| IBIS file stm32u595_599_5a5_5a9_wlcsp208_dsi_smps.ibs
[IBIS ver] 4.2
[File name] stm32u595_599_5a5_5a9_wlcsp208_dsi_smps.ibs
[File Rev] rev2.0
[Date]  11-09-2023
[Source] Data Created at STMicroelectronics
[Notes]  File originated from ELDO simulations.
[Disclaimer]  This information is for modeling purpose only and is
   not guaranteed. The information is subject to change without
   notice.
[Copyright] Copyright 2023 STMicroelectronics Inc.
|   Component stm32u595_599_5a5_5a9_wlcsp208_dsi_smps
[Component] stm32u595_599_5a5_5a9_wlcsp208_dsi_smps
[Manufacturer] STMicroelectronics
[Package]
| variable   typ   min   max
R_pkg  0  NA  NA
L_pkg  0  NA  NA
C_pkg  0  NA  NA
[Pin]   signal_name   model_name
A2  VDDUSB  power
A4  VDD11  nc
A6  VDD  power
A8  PA15  nc
A10  PD1  io8_100m_hslv_ft
A12  VDD  power
A14  PG13  io8_100m_hslv_ft
A16  VDDIO2  power
A18  PB6  io8_100m_i2c_ft
A20  PE0  io8_100m_hslv_ft
A22  VD11  nc
A24  VDD  power
A26  VDD  power
B1  PA12  io8_100m_ft
B3  PA13  io8_100m_ft
B5  VSS  gnd
B7  PH2  io8_100m_hslv_ft
B9  PC10  io8_100m_ft
B11  VSS  gnd
B13  PG9  io8_100m_hslv_ft
B15  VSS  gnd
B17  PB3  io8_100m_i2c_ft
B19  PB8  io8_100m_i2c_ft
B21  PE1  io8_100m_hslv_ft
B23  VSS  gnd
B25  VBAT  power
C2  PA11  io8_100m_ft
C4  PA10  io8_100m_usb_id
C6  PA9  io8_100m_usb_vbus_ft
C8  PA8  io8_166m_hslv_ft
C10  PC11  io8_100m_hslv_ft
C12  PD3  io8_166m_hslv_ft
C14  PD7  io8_100m_hslv_ft
C16  PG14  io8_100m_hslv_ft
C18  PB5  io8_166m_hslv_ft
C20  PB9  io8_100m_i2c_ft
C22  PI5  io8_100m_hslv_ft
C24  PE6  io8_100m_hslv_tamp_ft
C26  PC14-OSC32_IN  nc
D1  VDD11USB  nc
D3  PC7  io8_100m_ft
D5  PC6  io8_100m_ft
D7  PC8  io8_100m_ft
D9  PC9  io8_100m_ft
D11  PA14  io8_100m_ft
D13  PD2  io8_100m_ft
D15  PD4  io8_100m_hslv_ft
D17  PG12  io8_100m_hslv_ft
D19  PB7  io8_spi_hslv_ft
D21  PI6  io8_spi_ft
D23  PC13  io8_100m_ft
D25  PC15-OSC32_OUT  nc
E2  VDDIO2  power
E4  VSS  gnd
E6  PJ0  io8_spi_ft
E8  PI15  io8_spi_ft
E10  PH4  io8_100m_hslv_ft
E12  PH7  io8_spi_hslv_ft
E14  PC12  io8_166m_hslv_ft
E16  PD5  io8_100m_hslv_ft
E18  PG11  io8_100m_hslv_ft
E20  PH3-BOOT0  nc
E22  PE3  io8_100m_hslv_tamp_ft
E24  VSSDSI  nc
E26  DSI_D0P  nc
F1  VDD  power
F3  VSS  gnd
F5  PI14  io8_spi_ft
F7  PI13  io8_spi_ft
F9  PG2  io8_100m_hslv_ft
F11  PG8  io8_100m_i2c_ft
F13  PH5  io8_100m_i2c_ft
F15  PD0  io8_100m_hslv_ft
F17  PD6  io8_166m_hslv_ft
F19  PG10  io8_100m_hslv_ft
F21  PE4  io8_100m_hslv_tamp_ft
F23  VSS_DSI  nc
F25  DSI_D0N  nc
G2  VDD  power
G4  VSS  gnd
G6  PI11  io8_spi_ft
G8  PI12  io8_spi_ft
G10  PG6  io8_100m_hslv_ft
G12  PG5  io8_100m_hslv_ft
G14  PG7  io8_100m_hslv_ft
G16  PH8  io8_100m_hslv_ft
G18  PB4  io8_100m_i2c_ft
G20  PE2  io8_100m_hslv_ft
G22  PE5  io8_100m_hslv_tamp_ft
G24  VDDDSI  nc
G26  DSI_CKP  nc
H1  VDD  power
H3  VSS  gnd
H5  PI9  io8_spi_ft
H7  PI10  io8_spi_ft
H9  PG3  io8_100m_hslv_ft
H11  PG0  io8_100m_hslv_ft
H13  PB0  io8_100m_hslv_ft
H15  PH6  io8_166m_hslv_ft
H17  PG15  io8_100m_hslv_ft
H19  PF0  io8_100m_hslv_ft
H21  PF1  io8_100m_hslv_ft
H23  VSS_DSI  nc
H25  DSI_CKN  nc
J2  PI4  io8_spi_ft
J4  VSS  gnd
J6  PI2  io8_spi_ft
J8  PI8  io8_spi_ft
J10  PG4  io8_100m_hslv_ft
J12  PG1  io8_100m_hslv_ft
J14  PF7  io8_100m_hslv_ft
J16  PF6  io8_100m_hslv_ft
J18  PI7  io8_spi_ft
J20  PF2  io8_100m_hslv_ft
J22  PF4  io8_spi_ft
J24  VDD11DSI  nc
J26  DSI_D1P  nc
K1  PI3  io8_spi_ft
K3  VSS  gnd
K5  PI1  io8_spi_ft
K7  PI0  io8_spi_ft
K9  PD15  io8_100m_hslv_ft
K11  PD13  io8_100m_hslv_ft
K13  PF14  io8_100m_hslv_ft
K15  PC1  io8_spi_hslv_ft
K17  PC0  io8_100m_hslv_ft
K19  PF8  io8_100m_hslv_ft
K21  PF5  io8_spi_ft
K23  PF3  io8_100m_hslv_ft
K25  DSI_D1N  nc
L2  VDD  power
L4  VSS  gnd
L6  PH14  io8_spi_ft
L8  PH15  io8_spi_ft
L10  PD12  io8_100m_hslv_ft
L12  PE7  io8_100m_hslv_ft
L14  PB1  io8_100m_hslv_ft
L16  PA1  io8_100m_hslv_tamp_ft
L18  PC2  io8_100m_hslv_ft
L20  PF9  io8_100m_hslv_ft
L22  PF10  io8_166m_hslv_ft
L24  VSS  gnd
L26  VDD  power
M1  VDD  power
M3  VSS  gnd
M5  PH12  io8_spi_ft
M7  PH13  io8_spi_ft
M9  PH9  io8_spi_ft
M11  PD11  io8_100m_hslv_ft
M13  PE10  io8_166m_hslv_ft
M15  PB2  io8_100m_hslv_tamp_ft
M17  PA2  io8_100m_hslv_ft
M19  PC3  io8_100m_hslv_ft
M21  NRST  nc
M23  PH0-OSC_IN   nc
M25  PH1-OSC_OUT  nc
N2  VDD  power
N4  VSS  gnd
N6  PH10  io8_spi_ft
N8  PH11  io8_spi_ft
N10  PD14  io8_100m_hslv_ft
N12  PE13  io8_100m_hslv_ft
N14  PE8  io8_100m_hslv_ft
N16  PF11  io8_166m_hslv_ft
N18  PA6  io8_100m_hslv_ft
N20  PA4  io8_100m_hslv_ft
N22  PA0  io8_100m_hslv_tamp_ft
N24  VREFM  nc
N26  VSSA  nc
P1  VDD  power
P3  VSS  gnd
P5  PD10  io8_100m_hslv_ft
P7  PD9  io8_100m_hslv_ft
P9  PD8  io8_100m_hslv_ft
P11  PB15  nc
P13  PE14  io8_100m_hslv_ft
P15  PE11  io8_100m_hslv_ft
P17  PF13  io8_100m_hslv_ft
P19  PC5  io8_100m_tamp_ft
P21  PA5  io8_100m_ft
P23  PA3  io8_166m_hslv_ft
P25  VREFP  nc
R2  VDD  power
R4  VSS  gnd
R6  PB14  io8_100m_i2c_ft
R8  VSSSMPS  nc
R10  PB11  io8_100m_hslv_ft
R12  PE15  io8_100m_hslv_ft
R14  PE12  io8_100m_hslv_ft
R16  VSS  gnd
R18  PF15  io8_100m_hslv_ft
R20  VSS  gnd
R22  PA7  io8_100m_hslv_ft
R24  VSS  gnd
R26  VDDA  nc
T1  VDD  power
T3  VDD11  nc
T5  PB12  io8_166m_hslv_ft
T7  PB13  io8_100m_i2c_ft
T9  VDDSMPS  nc
T11  VLXSMPS  nc
T13  PB10  io8_spi_hslv_ft
T15  VDD  power
T17  PE9  io8_166m_hslv_ft
T19  VDD  power
T21  PF12  io8_100m_hslv_ft
T23  PC4  io8_100m_hslv_ft
T25  VDD  power
[Package Model]   481-wlcsp-208-221128
[Pin Mapping]   pulldown_ref   pullup_ref   | Comment
A2  nc  vddusb
A4  nc  nc
A6  nc  vddiom
A8  nc  nc
A10  gndio  vddiom
A12  nc  vddiom
A14  gndio  vddiom  | Depending on IO usage
| A14  gndio  vddio2  | Depending on IO usage
A16  nc  vddio2
A18  gndio  vddiom
A20  gndio  vddiom
A22  nc  nc
A24  nc  vddiom
A26  nc  vddiom
B1  gndio  vddiom  | Depending on IO usage
| B1  gndio  vddusb  | Depending on IO usage
B3  gndio  vddiom  | Depending on IO usage
| B3  gndio  vddusb  | Depending on IO usage
B5  gndio  nc
B7  gndio  vddiom
B9  gndio  vddiom
B11  gndio  nc
B13  gndio  vddiom  | Depending on IO usage
| B13  gndio  vddio2  | Depending on IO usage
B15  gndio  nc
B17  gndio  vddiom
B19  gndio  vddiom
B21  gndio  vddiom
B23  gndio  nc
B25  nc  vsw
C2  gndio  vddiom  | Depending on IO usage
| C2  gndio  vddusb  | Depending on IO usage
C4  gndio  vddiom  | Depending on IO usage
| C4  gndio  vddusb  | Depending on IO usage
C6  gndio  vddiom  | Depending on IO usage
| C6  gndio  vddusb  | Depending on IO usage
C8  gndio  vddiom
C10  gndio  vddiom
C12  gndio  vddiom
C14  gndio  vddiom
C16  gndio  vddiom  | Depending on IO usage
| C16  gndio  vddio2  | Depending on IO usage
C18  gndio  vddiom
C20  gndio  vddiom
C22  gndio  vddiom
C24  gndio  vddiom
C26  nc  nc
D1  nc  nc
D3  gndio  vddiom
D5  gndio  vddiom
D7  gndio  vddiom
D9  gndio  vddiom
D11  gndio  vddiom
D13  gndio  vddiom
D15  gndio  vddiom
D17  gndio  vddiom  | Depending on IO usage
| D17  gndio  vddio2  | Depending on IO usage
D19  gndio  vddiom
D21  gndio  vddiom
D23  gndio  vddiom  | Depending on IO usage
| D23  gndio  vsw  | Depending on IO usage
D25  nc  nc
E2  nc  vddio2
E4  gndio  nc
E6  gndio  vddiom
E8  gndio  vddiom
E10  gndio  vddiom
E12  gndio  vddiom
E14  gndio  vddiom
E16  gndio  vddiom
E18  gndio  vddiom  | Depending on IO usage
| E18  gndio  vddio2  | Depending on IO usage
E20  nc  nc
E22  gndio  vddiom
E24  nc  nc
E26  nc  nc
F1  nc  vddhspi
F3  gndio  nc
F5  gndio  vddiom
F7  gndio  vddiom
F9  gndio  vddiom  | Depending on IO usage
| F9  gndio  vddio2  | Depending on IO usage
F11  gndio  vddiom  | Depending on IO usage
| F11  gndio  vddio2  | Depending on IO usage
F13  gndio  vddiom
F15  gndio  vddiom
F17  gndio  vddiom
F19  gndio  vddiom  | Depending on IO usage
| F19  gndio  vddio2  | Depending on IO usage
F21  gndio  vddiom
F23  nc  nc
F25  nc  nc
G2  nc  vddhspi
G4  gndio  nc
G6  gndio  vddiom
G8  gndio  vddiom
G10  gndio  vddiom  | Depending on IO usage
| G10  gndio  vddio2  | Depending on IO usage
G12  gndio  vddiom  | Depending on IO usage
| G12  gndio  vddio2  | Depending on IO usage
G14  gndio  vddiom  | Depending on IO usage
| G14  gndio  vddio2  | Depending on IO usage
G16  gndio  vddiom
G18  gndio  vddiom
G20  gndio  vddiom
G22  gndio  vddiom
G24  nc  nc
G26  nc  nc
H1  nc  vddhspi
H3  gndio  nc
H5  gndio  vddiom
H7  gndio  vddiom
H9  gndio  vddiom  | Depending on IO usage
| H9  gndio  vddio2  | Depending on IO usage
H11  gndio  vddiom
H13  gndio  vddiom
H15  gndio  vddiom
H17  gndio  vddiom  | Depending on IO usage
| H17  gndio  vddio2  | Depending on IO usage
H19  gndio  vddiom
H21  gndio  vddiom
H23  nc  nc
H25  nc  nc
J2  gndio  vddiom
J4  gndio  nc
J6  gndio  vddiom
J8  gndio  vddiom
J10  gndio  vddiom  | Depending on IO usage
| J10  gndio  vddio2  | Depending on IO usage
J12  gndio  vddiom
J14  gndio  vddiom
J16  gndio  vddiom
J18  gndio  vddiom
J20  gndio  vddiom
J22  gndio  vddiom
J24  nc  nc
J26  nc  nc
K1  gndio  vddiom
K3  gndio  nc
K5  gndio  vddiom
K7  gndio  vddiom
K9  gndio  vddiom
K11  gndio  vddiom
K13  gndio  vddiom
K15  gndio  vddiom
K17  gndio  vddiom
K19  gndio  vddiom
K21  gndio  vddiom
K23  gndio  vddiom
K25  nc  nc
L2  nc  vddhspi
L4  gndio  nc
L6  gndio  vddiom
L8  gndio  vddiom
L10  gndio  vddiom
L12  gndio  vddiom
L14  gndio  vddiom
L16  gndio  vddiom
L18  gndio  vddiom
L20  gndio  vddiom
L22  gndio  vddiom
L24  gndio  nc
L26  nc  vddiom
M1  nc  vddhspi
M3  gndio  nc
M5  gndio  vddiom
M7  gndio  vddiom
M9  gndio  vddiom
M11  gndio  vddiom
M13  gndio  vddiom
M15  gndio  vddiom
M17  gndio  vddiom
M19  gndio  vddiom
M21  nc  nc
M23  nc  nc
M25  nc  nc
N2  nc  vddhspi
N4  gndio  nc
N6  gndio  vddiom
N8  gndio  vddiom
N10  gndio  vddiom
N12  gndio  vddiom
N14  gndio  vddiom
N16  gndio  vddiom
N18  gndio  vddiom
N20  gndio  vddiom
N22  gndio  vddiom
N24  nc  nc
N26  nc  nc
P1  nc  vddiom
P3  gndio  nc
P5  gndio  vddiom
P7  gndio  vddiom
P9  gndio  vddiom
P11  nc  nc
P13  gndio  vddiom
P15  gndio  vddiom
P17  gndio  vddiom
P19  gndio  vddiom
P21  gndio  vddiom
P23  gndio  vddiom
P25  nc  nc
R2  nc  vddiom
R4  gndio  nc
R6  gndio  vddiom
R8  nc  nc
R10  gndio  vddiom
R12  gndio  vddiom
R14  gndio  vddiom
R16  gndio  nc
R18  gndio  vddiom
R20  gndio  nc
R22  gndio  vddiom
R24  gndio  nc
R26  nc  nc
T1  nc  vddiom
T3  nc  nc
T5  gndio  vddiom
T7  gndio  vddiom
T9  nc  nc
T11  nc  nc
T13  gndio  vddiom
T15  nc  vddiom
T17  gndio  vddiom
T19  nc  vddiom
T21  gndio  vddiom
T23  gndio  vddiom
T25  nc  vddiom
[Model Selector] io8_100m_ft
io8_100m_ft_hs_1v2  "IO8_FT 100MHz high speed @ 1.2V"
io8_100m_ft_fs_1v2  "IO8_FT 100MHz fast speed @ 1.2V"
io8_100m_ft_fs_pd_1v2  "IO8_FT 100MHz fast speed @ 1.2V pulldown"
io8_100m_ft_ms_1v2  "IO8_FT 100MHz med speed @ 1.2V"
io8_100m_ft_ms_pd_1v2  "IO8_FT 100MHz med speed @ 1.2V pulldown"
io8_100m_ft_ls_1v2  "IO8_FT 100MHz low speed @ 1.2V"
io8_100m_ft_ls_pd_1v2  "IO8_FT 100MHz low speed @ 1.2V pulldown"
io8_100m_ft_hs_1v8  "IO8_FT 100MHz high speed @ 1.8V"
io8_100m_ft_hs_pd_1v8  "IO8_FT 100MHz high speed @ 1.8V pulldown"
io8_100m_ft_fs_1v8  "IO8_FT 100MHz fast speed @ 1.8V"
io8_100m_ft_fs_pd_1v8  "IO8_FT 100MHz fast speed @ 1.8V pulldown"
io8_100m_ft_ms_1v8  "IO8_FT 100MHz med speed @ 1.8V"
io8_100m_ft_ms_pd_1v8  "IO8_FT 100MHz med speed @ 1.8V pulldown"
io8_100m_ft_ls_1v8  "IO8_FT 100MHz low speed @ 1.8V"
io8_100m_ft_ls_pd_1v8  "IO8_FT 100MHz low speed @ 1.8V pulldown"
io8_100m_ft_hs_3v3  "IO8_FT 100MHz high speed @ 3.3V"
io8_100m_ft_hs_pd_3v3  "IO8_FT 100MHz high speed @ 3.3V pulldown"
io8_100m_ft_fs_3v3  "IO8_FT 100MHz fast speed @ 3.3V"
io8_100m_ft_fs_pd_3v3  "IO8_FT 100MHz fast speed @ 3.3V pulldown"
io8_100m_ft_ms_3v3  "IO8_FT 100MHz med speed @ 3.3V"
io8_100m_ft_ms_pd_3v3  "IO8_FT 100MHz med speed @ 3.3V pulldown"
io8_100m_ft_ls_3v3  "IO8_FT 100MHz low speed @ 3.3V"
io8_100m_ft_ls_pd_3v3  "IO8_FT 100MHz low speed @ 3.3V pulldown"
[Model Selector] io8_100m_hslv_ft
io8_100m_ft_hs_1v2  "IO8_FT 100MHz high speed @ 1.2V"
io8_100m_ft_hs_pu_1v2  "IO8_FT 100MHz high speed @ 1.2V pullup"
io8_100m_ft_hs_pd_1v2  "IO8_FT 100MHz high speed @ 1.2V pulldown"
io8_100m_ft_fs_1v2  "IO8_FT 100MHz fast speed @ 1.2V"
io8_100m_ft_fs_pu_1v2  "IO8_FT 100MHz fast speed @ 1.2V pullup"
io8_100m_ft_fs_pd_1v2  "IO8_FT 100MHz fast speed @ 1.2V pulldown"
io8_100m_ft_ms_1v2  "IO8_FT 100MHz med speed @ 1.2V"
io8_100m_ft_ms_pu_1v2  "IO8_FT 100MHz med speed @ 1.2V pullup"
io8_100m_ft_ms_pd_1v2  "IO8_FT 100MHz med speed @ 1.2V pulldown"
io8_100m_ft_ls_1v2  "IO8_FT 100MHz low speed @ 1.2V"
io8_100m_ft_ls_pu_1v2  "IO8_FT 100MHz low speed @ 1.2V pullup"
io8_100m_ft_ls_pd_1v2  "IO8_FT 100MHz low speed @ 1.2V pulldown"
io8_100m_ft_hs_1v8  "IO8_FT 100MHz high speed @ 1.8V"
io8_100m_ft_hs_pu_1v8  "IO8_FT 100MHz high speed @ 1.8V pullup"
io8_100m_ft_hs_pd_1v8  "IO8_FT 100MHz high speed @ 1.8V pulldown"
io8_100m_ft_fs_1v8  "IO8_FT 100MHz fast speed @ 1.8V"
io8_100m_ft_fs_pu_1v8  "IO8_FT 100MHz fast speed @ 1.8V pullup"
io8_100m_ft_fs_pd_1v8  "IO8_FT 100MHz fast speed @ 1.8V pulldown"
io8_100m_ft_ms_1v8  "IO8_FT 100MHz med speed @ 1.8V"
io8_100m_ft_ms_pu_1v8  "IO8_FT 100MHz med speed @ 1.8V pullup"
io8_100m_ft_ms_pd_1v8  "IO8_FT 100MHz med speed @ 1.8V pulldown"
io8_100m_ft_ls_1v8  "IO8_FT 100MHz low speed @ 1.8V"
io8_100m_ft_ls_pu_1v8  "IO8_FT 100MHz low speed @ 1.8V pullup"
io8_100m_ft_ls_pd_1v8  "IO8_FT 100MHz low speed @ 1.8V pulldown"
io8_100m_ft_hs_3v3  "IO8_FT 100MHz high speed @ 3.3V"
io8_100m_ft_hs_pu_3v3  "IO8_FT 100MHz high speed @ 3.3V pullup"
io8_100m_ft_hs_pd_3v3  "IO8_FT 100MHz high speed @ 3.3V pulldown"
io8_100m_ft_fs_3v3  "IO8_FT 100MHz fast speed @ 3.3V"
io8_100m_ft_fs_pu_3v3  "IO8_FT 100MHz fast speed @ 3.3V pullup"
io8_100m_ft_fs_pd_3v3  "IO8_FT 100MHz fast speed @ 3.3V pulldown"
io8_100m_ft_ms_3v3  "IO8_FT 100MHz med speed @ 3.3V"
io8_100m_ft_ms_pu_3v3  "IO8_FT 100MHz med speed @ 3.3V pullup"
io8_100m_ft_ms_pd_3v3  "IO8_FT 100MHz med speed @ 3.3V pulldown"
io8_100m_ft_ls_3v3  "IO8_FT 100MHz low speed @ 3.3V"
io8_100m_ft_ls_pu_3v3  "IO8_FT 100MHz low speed @ 3.3V pullup"
io8_100m_ft_ls_pd_3v3  "IO8_FT 100MHz low speed @ 3.3V pulldown"
io8_100m_hslv_ft_hs_1v2  "IO8_FT 100MHz HSLV high speed @ 1.2V"
io8_100m_hslv_ft_hs_pu_1v2  "IO8_FT 100MHz HSLV high speed @ 1.2V pullup"
io8_100m_hslv_ft_hs_pd_1v2  "IO8_FT 100MHz HSLV high speed @ 1.2V pulldown"
io8_100m_hslv_ft_fs_1v2  "IO8_FT 100MHz HSLV fast speed @ 1.2V"
io8_100m_hslv_ft_fs_pu_1v2  "IO8_FT 100MHz HSLV fast speed @ 1.2V pullup"
io8_100m_hslv_ft_fs_pd_1v2  "IO8_FT 100MHz HSLV fast speed @ 1.2V pulldown"
io8_100m_hslv_ft_ms_1v2  "IO8_FT 100MHz HSLV med speed @ 1.2V"
io8_100m_hslv_ft_ms_pu_1v2  "IO8_FT 100MHz HSLV med speed @ 1.2V pullup"
io8_100m_hslv_ft_ms_pd_1v2  "IO8_FT 100MHz HSLV med speed @ 1.2V pulldown"
io8_100m_hslv_ft_ls_1v2  "IO8_FT 100MHz HSLV low speed @ 1.2V"
io8_100m_hslv_ft_ls_pu_1v2  "IO8_FT 100MHz HSLV low speed @ 1.2V pullup"
io8_100m_hslv_ft_ls_pd_1v2  "IO8_FT 100MHz HSLV low speed @ 1.2V pulldown"
io8_100m_hslv_ft_hs_1v8  "IO8_FT 100MHz HSLV high speed @ 1.8V"
io8_100m_hslv_ft_hs_pu_1v8  "IO8_FT 100MHz HSLV high speed @ 1.8V pullup"
io8_100m_hslv_ft_hs_pd_1v8  "IO8_FT 100MHz HSLV high speed @ 1.8V pulldown"
io8_100m_hslv_ft_fs_1v8  "IO8_FT 100MHz HSLV fast speed @ 1.8V"
io8_100m_hslv_ft_fs_pu_1v8  "IO8_FT 100MHz HSLV fast speed @ 1.8V pullup"
io8_100m_hslv_ft_fs_pd_1v8  "IO8_FT 100MHz HSLV fast speed @ 1.8V pulldown"
io8_100m_hslv_ft_ms_1v8  "IO8_FT 100MHz HSLV med speed @ 1.8V"
io8_100m_hslv_ft_ms_pu_1v8  "IO8_FT 100MHz HSLV med speed @ 1.8V pullup"
io8_100m_hslv_ft_ms_pd_1v8  "IO8_FT 100MHz HSLV med speed @ 1.8V pulldown"
io8_100m_hslv_ft_ls_1v8  "IO8_FT 100MHz HSLV low speed @ 1.8V"
io8_100m_hslv_ft_ls_pu_1v8  "IO8_FT 100MHz HSLV low speed @ 1.8V pullup"
io8_100m_hslv_ft_ls_pd_1v8  "IO8_FT 100MHz HSLV low speed @ 1.8V pulldown"
io8_100m_hslv_ft_hs_2v5  "IO8_FT 100MHz HSLV high speed @ 2.5V"
io8_100m_hslv_ft_hs_pu_2v5  "IO8_FT 100MHz HSLV high speed @ 2.5V pullup"
io8_100m_hslv_ft_hs_pd_2v5  "IO8_FT 100MHz HSLV high speed @ 2.5V pulldown"
io8_100m_hslv_ft_fs_2v5  "IO8_FT 100MHz HSLV fast speed @ 2.5V"
io8_100m_hslv_ft_fs_pu_2v5  "IO8_FT 100MHz HSLV fast speed @ 2.5V pullup"
io8_100m_hslv_ft_fs_pd_2v5  "IO8_FT 100MHz HSLV fast speed @ 2.5V pulldown"
io8_100m_hslv_ft_ms_2v5  "IO8_FT 100MHz HSLV med speed @ 2.5V"
io8_100m_hslv_ft_ms_pu_2v5  "IO8_FT 100MHz HSLV med speed @ 2.5V pullup"
io8_100m_hslv_ft_ms_pd_2v5  "IO8_FT 100MHz HSLV med speed @ 2.5V pulldown"
io8_100m_hslv_ft_ls_2v5  "IO8_FT 100MHz HSLV low speed @ 2.5V"
io8_100m_hslv_ft_ls_pu_2v5  "IO8_FT 100MHz HSLV low speed @ 2.5V pullup"
io8_100m_hslv_ft_ls_pd_2v5  "IO8_FT 100MHz HSLV low speed @ 2.5V pulldown"
[Model Selector] io8_100m_hslv_tamp_ft
io8_100m_ft_hs_1v2  "IO8_FT 100MHz high speed @ 1.2V"
io8_100m_ft_hs_pu_1v2  "IO8_FT 100MHz high speed @ 1.2V pullup"
io8_100m_ft_hs_pd_1v2  "IO8_FT 100MHz high speed @ 1.2V pulldown"
io8_100m_ft_fs_1v2  "IO8_FT 100MHz fast speed @ 1.2V"
io8_100m_ft_fs_pu_1v2  "IO8_FT 100MHz fast speed @ 1.2V pullup"
io8_100m_ft_fs_pd_1v2  "IO8_FT 100MHz fast speed @ 1.2V pulldown"
io8_100m_ft_ms_1v2  "IO8_FT 100MHz med speed @ 1.2V"
io8_100m_ft_ms_pu_1v2  "IO8_FT 100MHz med speed @ 1.2V pullup"
io8_100m_ft_ms_pd_1v2  "IO8_FT 100MHz med speed @ 1.2V pulldown"
io8_100m_ft_ls_1v2  "IO8_FT 100MHz low speed @ 1.2V"
io8_100m_ft_ls_pu_1v2  "IO8_FT 100MHz low speed @ 1.2V pullup"
io8_100m_ft_ls_pd_1v2  "IO8_FT 100MHz low speed @ 1.2V pulldown"
io8_100m_ft_hs_1v8  "IO8_FT 100MHz high speed @ 1.8V"
io8_100m_ft_hs_pu_1v8  "IO8_FT 100MHz high speed @ 1.8V pullup"
io8_100m_ft_hs_pd_1v8  "IO8_FT 100MHz high speed @ 1.8V pulldown"
io8_100m_ft_fs_1v8  "IO8_FT 100MHz fast speed @ 1.8V"
io8_100m_ft_fs_pu_1v8  "IO8_FT 100MHz fast speed @ 1.8V pullup"
io8_100m_ft_fs_pd_1v8  "IO8_FT 100MHz fast speed @ 1.8V pulldown"
io8_100m_ft_ms_1v8  "IO8_FT 100MHz med speed @ 1.8V"
io8_100m_ft_ms_pu_1v8  "IO8_FT 100MHz med speed @ 1.8V pullup"
io8_100m_ft_ms_pd_1v8  "IO8_FT 100MHz med speed @ 1.8V pulldown"
io8_100m_ft_ls_1v8  "IO8_FT 100MHz low speed @ 1.8V"
io8_100m_ft_ls_pu_1v8  "IO8_FT 100MHz low speed @ 1.8V pullup"
io8_100m_ft_ls_pd_1v8  "IO8_FT 100MHz low speed @ 1.8V pulldown"
io8_100m_ft_hs_3v3  "IO8_FT 100MHz high speed @ 3.3V"
io8_100m_ft_hs_pu_3v3  "IO8_FT 100MHz high speed @ 3.3V pullup"
io8_100m_ft_hs_pd_3v3  "IO8_FT 100MHz high speed @ 3.3V pulldown"
io8_100m_ft_fs_3v3  "IO8_FT 100MHz fast speed @ 3.3V"
io8_100m_ft_fs_pu_3v3  "IO8_FT 100MHz fast speed @ 3.3V pullup"
io8_100m_ft_fs_pd_3v3  "IO8_FT 100MHz fast speed @ 3.3V pulldown"
io8_100m_ft_ms_3v3  "IO8_FT 100MHz med speed @ 3.3V"
io8_100m_ft_ms_pu_3v3  "IO8_FT 100MHz med speed @ 3.3V pullup"
io8_100m_ft_ms_pd_3v3  "IO8_FT 100MHz med speed @ 3.3V pulldown"
io8_100m_ft_ls_3v3  "IO8_FT 100MHz low speed @ 3.3V"
io8_100m_ft_ls_pu_3v3  "IO8_FT 100MHz low speed @ 3.3V pullup"
io8_100m_ft_ls_pd_3v3  "IO8_FT 100MHz low speed @ 3.3V pulldown"
io8_100m_hslv_ft_hs_1v2  "IO8_FT 100MHz HSLV high speed @ 1.2V"
io8_100m_hslv_ft_hs_pu_1v2  "IO8_FT 100MHz HSLV high speed @ 1.2V pullup"
io8_100m_hslv_ft_hs_pd_1v2  "IO8_FT 100MHz HSLV high speed @ 1.2V pulldown"
io8_100m_hslv_ft_fs_1v2  "IO8_FT 100MHz HSLV fast speed @ 1.2V"
io8_100m_hslv_ft_fs_pu_1v2  "IO8_FT 100MHz HSLV fast speed @ 1.2V pullup"
io8_100m_hslv_ft_fs_pd_1v2  "IO8_FT 100MHz HSLV fast speed @ 1.2V pulldown"
io8_100m_hslv_ft_ms_1v2  "IO8_FT 100MHz HSLV med speed @ 1.2V"
io8_100m_hslv_ft_ms_pu_1v2  "IO8_FT 100MHz HSLV med speed @ 1.2V pullup"
io8_100m_hslv_ft_ms_pd_1v2  "IO8_FT 100MHz HSLV med speed @ 1.2V pulldown"
io8_100m_hslv_ft_ls_1v2  "IO8_FT 100MHz HSLV low speed @ 1.2V"
io8_100m_hslv_ft_ls_pu_1v2  "IO8_FT 100MHz HSLV low speed @ 1.2V pullup"
io8_100m_hslv_ft_ls_pd_1v2  "IO8_FT 100MHz HSLV low speed @ 1.2V pulldown"
io8_100m_hslv_ft_hs_1v8  "IO8_FT 100MHz HSLV high speed @ 1.8V"
io8_100m_hslv_ft_hs_pu_1v8  "IO8_FT 100MHz HSLV high speed @ 1.8V pullup"
io8_100m_hslv_ft_hs_pd_1v8  "IO8_FT 100MHz HSLV high speed @ 1.8V pulldown"
io8_100m_hslv_ft_fs_1v8  "IO8_FT 100MHz HSLV fast speed @ 1.8V"
io8_100m_hslv_ft_fs_pu_1v8  "IO8_FT 100MHz HSLV fast speed @ 1.8V pullup"
io8_100m_hslv_ft_fs_pd_1v8  "IO8_FT 100MHz HSLV fast speed @ 1.8V pulldown"
io8_100m_hslv_ft_ms_1v8  "IO8_FT 100MHz HSLV med speed @ 1.8V"
io8_100m_hslv_ft_ms_pu_1v8  "IO8_FT 100MHz HSLV med speed @ 1.8V pullup"
io8_100m_hslv_ft_ms_pd_1v8  "IO8_FT 100MHz HSLV med speed @ 1.8V pulldown"
io8_100m_hslv_ft_ls_1v8  "IO8_FT 100MHz HSLV low speed @ 1.8V"
io8_100m_hslv_ft_ls_pu_1v8  "IO8_FT 100MHz HSLV low speed @ 1.8V pullup"
io8_100m_hslv_ft_ls_pd_1v8  "IO8_FT 100MHz HSLV low speed @ 1.8V pulldown"
io8_100m_hslv_ft_hs_2v5  "IO8_FT 100MHz HSLV high speed @ 2.5V"
io8_100m_hslv_ft_hs_pu_2v5  "IO8_FT 100MHz HSLV high speed @ 2.5V pullup"
io8_100m_hslv_ft_hs_pd_2v5  "IO8_FT 100MHz HSLV high speed @ 2.5V pulldown"
io8_100m_hslv_ft_fs_2v5  "IO8_FT 100MHz HSLV fast speed @ 2.5V"
io8_100m_hslv_ft_fs_pu_2v5  "IO8_FT 100MHz HSLV fast speed @ 2.5V pullup"
io8_100m_hslv_ft_fs_pd_2v5  "IO8_FT 100MHz HSLV fast speed @ 2.5V pulldown"
io8_100m_hslv_ft_ms_2v5  "IO8_FT 100MHz HSLV med speed @ 2.5V"
io8_100m_hslv_ft_ms_pu_2v5  "IO8_FT 100MHz HSLV med speed @ 2.5V pullup"
io8_100m_hslv_ft_ms_pd_2v5  "IO8_FT 100MHz HSLV med speed @ 2.5V pulldown"
io8_100m_hslv_ft_ls_2v5  "IO8_FT 100MHz HSLV low speed @ 2.5V"
io8_100m_hslv_ft_ls_pu_2v5  "IO8_FT 100MHz HSLV low speed @ 2.5V pullup"
io8_100m_hslv_ft_ls_pd_2v5  "IO8_FT 100MHz HSLV low speed @ 2.5V pulldown"
io8_ft_v33_hs_1v2  "IO8_FT_V33 high speed @ 1.2V"
io8_ft_v33_hs_pu_1v2  "IO8_FT_V33 high speed @ 1.2V pullup"
io8_ft_v33_hs_pd_1v2  "IO8_FT_V33 high speed @ 1.2V pulldown"
io8_ft_v33_fs_1v2  "IO8_FT_V33 fast speed @ 1.2V"
io8_ft_v33_fs_pu_1v2  "IO8_FT_V33 fast speed @ 1.2V pullup"
io8_ft_v33_fs_pd_1v2  "IO8_FT_V33 fast speed @ 1.2V pulldown"
io8_ft_v33_ms_1v2  "IO8_FT_V33 med speed @ 1.2V"
io8_ft_v33_ms_pu_1v2  "IO8_FT_V33 med speed @ 1.2V pullup"
io8_ft_v33_ms_pd_1v2  "IO8_FT_V33 med speed @ 1.2V pulldown"
io8_ft_v33_ls_1v2  "IO8_FT_V33 low speed @ 1.2V"
io8_ft_v33_ls_pu_1v2  "IO8_FT_V33 low speed @ 1.2V pullup"
io8_ft_v33_ls_pd_1v2  "IO8_FT_V33 low speed @ 1.2V pulldown"
io8_ft_v33_hs_1v8  "IO8_FT_V33 high speed @ 1.8V"
io8_ft_v33_hs_pu_1v8  "IO8_FT_V33 high speed @ 1.8V pullup"
io8_ft_v33_hs_pd_1v8  "IO8_FT_V33 high speed @ 1.8V pulldown"
io8_ft_v33_fs_1v8  "IO8_FT_V33 fast speed @ 1.8V"
io8_ft_v33_fs_pu_1v8  "IO8_FT_V33 fast speed @ 1.8V pullup"
io8_ft_v33_fs_pd_1v8  "IO8_FT_V33 fast speed @ 1.8V pulldown"
io8_ft_v33_ms_1v8  "IO8_FT_V33 med speed @ 1.8V"
io8_ft_v33_ms_pu_1v8  "IO8_FT_V33 med speed @ 1.8V pullup"
io8_ft_v33_ms_pd_1v8  "IO8_FT_V33 med speed @ 1.8V pulldown"
io8_ft_v33_ls_1v8  "IO8_FT_V33 low speed @ 1.8V"
io8_ft_v33_ls_pu_1v8  "IO8_FT_V33 low speed @ 1.8V pullup"
io8_ft_v33_ls_pd_1v8  "IO8_FT_V33 low speed @ 1.8V pulldown"
io8_ft_v33_hs_3v3  "IO8_FT_V33 high speed @ 3.3V"
io8_ft_v33_hs_pu_3v3  "IO8_FT_V33 high speed @ 3.3V pullup"
io8_ft_v33_hs_pd_3v3  "IO8_FT_V33 high speed @ 3.3V pulldown"
io8_ft_v33_fs_3v3  "IO8_FT_V33 fast speed @ 3.3V"
io8_ft_v33_fs_pu_3v3  "IO8_FT_V33 fast speed @ 3.3V pullup"
io8_ft_v33_fs_pd_3v3  "IO8_FT_V33 fast speed @ 3.3V pulldown"
io8_ft_v33_ms_3v3  "IO8_FT_V33 med speed @ 3.3V"
io8_ft_v33_ms_pu_3v3  "IO8_FT_V33 med speed @ 3.3V pullup"
io8_ft_v33_ms_pd_3v3  "IO8_FT_V33 med speed @ 3.3V pulldown"
io8_ft_v33_ls_3v3  "IO8_FT_V33 low speed @ 3.3V"
io8_ft_v33_ls_pu_3v3  "IO8_FT_V33 low speed @ 3.3V pullup"
io8_ft_v33_ls_pd_3v3  "IO8_FT_V33 low speed @ 3.3V pulldown"
[Model Selector] io8_100m_i2c_ft
io8_100m_ft_hs_1v2  "IO8_FT 100MHz high speed @ 1.2V"
io8_100m_ft_hs_pu_1v2  "IO8_FT 100MHz high speed @ 1.2V pullup"
io8_100m_ft_hs_pd_1v2  "IO8_FT 100MHz high speed @ 1.2V pulldown"
io8_100m_ft_fs_1v2  "IO8_FT 100MHz fast speed @ 1.2V"
io8_100m_ft_fs_pu_1v2  "IO8_FT 100MHz fast speed @ 1.2V pullup"
io8_100m_ft_fs_pd_1v2  "IO8_FT 100MHz fast speed @ 1.2V pulldown"
io8_100m_ft_ms_1v2  "IO8_FT 100MHz med speed @ 1.2V"
io8_100m_ft_ms_pu_1v2  "IO8_FT 100MHz med speed @ 1.2V pullup"
io8_100m_ft_ms_pd_1v2  "IO8_FT 100MHz med speed @ 1.2V pulldown"
io8_100m_ft_ls_1v2  "IO8_FT 100MHz low speed @ 1.2V"
io8_100m_ft_ls_pu_1v2  "IO8_FT 100MHz low speed @ 1.2V pullup"
io8_100m_ft_ls_pd_1v2  "IO8_FT 100MHz low speed @ 1.2V pulldown"
io8_100m_ft_hs_1v8  "IO8_FT 100MHz high speed @ 1.8V"
io8_100m_ft_hs_pu_1v8  "IO8_FT 100MHz high speed @ 1.8V pullup"
io8_100m_ft_hs_pd_1v8  "IO8_FT 100MHz high speed @ 1.8V pulldown"
io8_100m_ft_fs_1v8  "IO8_FT 100MHz fast speed @ 1.8V"
io8_100m_ft_fs_pu_1v8  "IO8_FT 100MHz fast speed @ 1.8V pullup"
io8_100m_ft_fs_pd_1v8  "IO8_FT 100MHz fast speed @ 1.8V pulldown"
io8_100m_ft_ms_1v8  "IO8_FT 100MHz med speed @ 1.8V"
io8_100m_ft_ms_pu_1v8  "IO8_FT 100MHz med speed @ 1.8V pullup"
io8_100m_ft_ms_pd_1v8  "IO8_FT 100MHz med speed @ 1.8V pulldown"
io8_100m_ft_ls_1v8  "IO8_FT 100MHz low speed @ 1.8V"
io8_100m_ft_ls_pu_1v8  "IO8_FT 100MHz low speed @ 1.8V pullup"
io8_100m_ft_ls_pd_1v8  "IO8_FT 100MHz low speed @ 1.8V pulldown"
io8_100m_ft_hs_3v3  "IO8_FT 100MHz high speed @ 3.3V"
io8_100m_ft_hs_pu_3v3  "IO8_FT 100MHz high speed @ 3.3V pullup"
io8_100m_ft_hs_pd_3v3  "IO8_FT 100MHz high speed @ 3.3V pulldown"
io8_100m_ft_fs_3v3  "IO8_FT 100MHz fast speed @ 3.3V"
io8_100m_ft_fs_pu_3v3  "IO8_FT 100MHz fast speed @ 3.3V pullup"
io8_100m_ft_fs_pd_3v3  "IO8_FT 100MHz fast speed @ 3.3V pulldown"
io8_100m_ft_ms_3v3  "IO8_FT 100MHz med speed @ 3.3V"
io8_100m_ft_ms_pu_3v3  "IO8_FT 100MHz med speed @ 3.3V pullup"
io8_100m_ft_ms_pd_3v3  "IO8_FT 100MHz med speed @ 3.3V pulldown"
io8_100m_ft_ls_3v3  "IO8_FT 100MHz low speed @ 3.3V"
io8_100m_ft_ls_pu_3v3  "IO8_FT 100MHz low speed @ 3.3V pullup"
io8_100m_ft_ls_pd_3v3  "IO8_FT 100MHz low speed @ 3.3V pulldown"
io8_100m_i2c_ft_1v2  "IO8_FT 100MHz I2C @ 1.2V"
io8_100m_i2c_ft_pu_1v2  "IO8_FT 100MHz I2C @ 1.2V pullup"
io8_100m_i2c_ft_pd_1v2  "IO8_FT 100MHz I2C @ 1.2V pulldown"
io8_100m_i2c_ft_1v8  "IO8_FT 100MHz I2C @ 1.8V"
io8_100m_i2c_ft_pu_1v8  "IO8_FT 100MHz I2C @ 1.8V pullup"
io8_100m_i2c_ft_pd_1v8  "IO8_FT 100MHz I2C @ 1,8V pulldown"
io8_100m_i2c_ft_3v3  "IO8_FT 100MHz I2C @ 3.3V"
io8_100m_i2c_ft_pu_3v3  "IO8_FT 100MHz I2C HSLV @ 3.3V pullup"
io8_100m_i2c_ft_pd_3v3  "IO8_FT 100MHz I2C @ 3.3V pulldown"
[Model Selector] io8_100m_tamp_ft
io8_100m_ft_hs_1v2  "IO8_FT 100MHz high speed @ 1.2V"
io8_100m_ft_hs_pu_1v2  "IO8_FT 100MHz high speed @ 1.2V pullup"
io8_100m_ft_hs_pd_1v2  "IO8_FT 100MHz high speed @ 1.2V pulldown"
io8_100m_ft_fs_1v2  "IO8_FT 100MHz fast speed @ 1.2V"
io8_100m_ft_fs_pu_1v2  "IO8_FT 100MHz fast speed @ 1.2V pullup"
io8_100m_ft_fs_pd_1v2  "IO8_FT 100MHz fast speed @ 1.2V pulldown"
io8_100m_ft_ms_1v2  "IO8_FT 100MHz med speed @ 1.2V"
io8_100m_ft_ms_pu_1v2  "IO8_FT 100MHz med speed @ 1.2V pullup"
io8_100m_ft_ms_pd_1v2  "IO8_FT 100MHz med speed @ 1.2V pulldown"
io8_100m_ft_ls_1v2  "IO8_FT 100MHz low speed @ 1.2V"
io8_100m_ft_ls_pu_1v2  "IO8_FT 100MHz low speed @ 1.2V pullup"
io8_100m_ft_ls_pd_1v2  "IO8_FT 100MHz low speed @ 1.2V pulldown"
io8_100m_ft_hs_1v8  "IO8_FT 100MHz high speed @ 1.8V"
io8_100m_ft_hs_pu_1v8  "IO8_FT 100MHz high speed @ 1.8V pullup"
io8_100m_ft_hs_pd_1v8  "IO8_FT 100MHz high speed @ 1.8V pulldown"
io8_100m_ft_fs_1v8  "IO8_FT 100MHz fast speed @ 1.8V"
io8_100m_ft_fs_pu_1v8  "IO8_FT 100MHz fast speed @ 1.8V pullup"
io8_100m_ft_fs_pd_1v8  "IO8_FT 100MHz fast speed @ 1.8V pulldown"
io8_100m_ft_ms_1v8  "IO8_FT 100MHz med speed @ 1.8V"
io8_100m_ft_ms_pu_1v8  "IO8_FT 100MHz med speed @ 1.8V pullup"
io8_100m_ft_ms_pd_1v8  "IO8_FT 100MHz med speed @ 1.8V pulldown"
io8_100m_ft_ls_1v8  "IO8_FT 100MHz low speed @ 1.8V"
io8_100m_ft_ls_pu_1v8  "IO8_FT 100MHz low speed @ 1.8V pullup"
io8_100m_ft_ls_pd_1v8  "IO8_FT 100MHz low speed @ 1.8V pulldown"
io8_100m_ft_hs_3v3  "IO8_FT 100MHz high speed @ 3.3V"
io8_100m_ft_hs_pu_3v3  "IO8_FT 100MHz high speed @ 3.3V pullup"
io8_100m_ft_hs_pd_3v3  "IO8_FT 100MHz high speed @ 3.3V pulldown"
io8_100m_ft_fs_3v3  "IO8_FT 100MHz fast speed @ 3.3V"
io8_100m_ft_fs_pu_3v3  "IO8_FT 100MHz fast speed @ 3.3V pullup"
io8_100m_ft_fs_pd_3v3  "IO8_FT 100MHz fast speed @ 3.3V pulldown"
io8_100m_ft_ms_3v3  "IO8_FT 100MHz med speed @ 3.3V"
io8_100m_ft_ms_pu_3v3  "IO8_FT 100MHz med speed @ 3.3V pullup"
io8_100m_ft_ms_pd_3v3  "IO8_FT 100MHz med speed @ 3.3V pulldown"
io8_100m_ft_ls_3v3  "IO8_FT 100MHz low speed @ 3.3V"
io8_100m_ft_ls_pu_3v3  "IO8_FT 100MHz low speed @ 3.3V pullup"
io8_100m_ft_ls_pd_3v3  "IO8_FT 100MHz low speed @ 3.3V pulldown"
io8_ft_v33_hs_1v2  "IO8_FT_V33 high speed @ 1.2V"
io8_ft_v33_hs_pu_1v2  "IO8_FT_V33 high speed @ 1.2V pullup"
io8_ft_v33_hs_pd_1v2  "IO8_FT_V33 high speed @ 1.2V pulldown"
io8_ft_v33_fs_1v2  "IO8_FT_V33 fast speed @ 1.2V"
io8_ft_v33_fs_pu_1v2  "IO8_FT_V33 fast speed @ 1.2V pullup"
io8_ft_v33_fs_pd_1v2  "IO8_FT_V33 fast speed @ 1.2V pulldown"
io8_ft_v33_ms_1v2  "IO8_FT_V33 med speed @ 1.2V"
io8_ft_v33_ms_pu_1v2  "IO8_FT_V33 med speed @ 1.2V pullup"
io8_ft_v33_ms_pd_1v2  "IO8_FT_V33 med speed @ 1.2V pulldown"
io8_ft_v33_ls_1v2  "IO8_FT_V33 low speed @ 1.2V"
io8_ft_v33_ls_pu_1v2  "IO8_FT_V33 low speed @ 1.2V pullup"
io8_ft_v33_ls_pd_1v2  "IO8_FT_V33 low speed @ 1.2V pulldown"
io8_ft_v33_hs_1v8  "IO8_FT_V33 high speed @ 1.8V"
io8_ft_v33_hs_pu_1v8  "IO8_FT_V33 high speed @ 1.8V pullup"
io8_ft_v33_hs_pd_1v8  "IO8_FT_V33 high speed @ 1.8V pulldown"
io8_ft_v33_fs_1v8  "IO8_FT_V33 fast speed @ 1.8V"
io8_ft_v33_fs_pu_1v8  "IO8_FT_V33 fast speed @ 1.8V pullup"
io8_ft_v33_fs_pd_1v8  "IO8_FT_V33 fast speed @ 1.8V pulldown"
io8_ft_v33_ms_1v8  "IO8_FT_V33 med speed @ 1.8V"
io8_ft_v33_ms_pu_1v8  "IO8_FT_V33 med speed @ 1.8V pullup"
io8_ft_v33_ms_pd_1v8  "IO8_FT_V33 med speed @ 1.8V pulldown"
io8_ft_v33_ls_1v8  "IO8_FT_V33 low speed @ 1.8V"
io8_ft_v33_ls_pu_1v8  "IO8_FT_V33 low speed @ 1.8V pullup"
io8_ft_v33_ls_pd_1v8  "IO8_FT_V33 low speed @ 1.8V pulldown"
io8_ft_v33_hs_3v3  "IO8_FT_V33 high speed @ 3.3V"
io8_ft_v33_hs_pu_3v3  "IO8_FT_V33 high speed @ 3.3V pullup"
io8_ft_v33_hs_pd_3v3  "IO8_FT_V33 high speed @ 3.3V pulldown"
io8_ft_v33_fs_3v3  "IO8_FT_V33 fast speed @ 3.3V"
io8_ft_v33_fs_pu_3v3  "IO8_FT_V33 fast speed @ 3.3V pullup"
io8_ft_v33_fs_pd_3v3  "IO8_FT_V33 fast speed @ 3.3V pulldown"
io8_ft_v33_ms_3v3  "IO8_FT_V33 med speed @ 3.3V"
io8_ft_v33_ms_pu_3v3  "IO8_FT_V33 med speed @ 3.3V pullup"
io8_ft_v33_ms_pd_3v3  "IO8_FT_V33 med speed @ 3.3V pulldown"
io8_ft_v33_ls_3v3  "IO8_FT_V33 low speed @ 3.3V"
io8_ft_v33_ls_pu_3v3  "IO8_FT_V33 low speed @ 3.3V pullup"
io8_ft_v33_ls_pd_3v3  "IO8_FT_V33 low speed @ 3.3V pulldown"
[Model Selector] io8_100m_usb_id
io8_100m_ft_hs_1v2  "IO8_FT 100MHz high speed @ 1.2V"
io8_100m_ft_hs_pu_1v2  "IO8_FT 100MHz high speed @ 1.2V pullup"
io8_100m_ft_hs_pd_1v2  "IO8_FT 100MHz high speed @ 1.2V pulldown"
io8_100m_ft_fs_1v2  "IO8_FT 100MHz fast speed @ 1.2V"
io8_100m_ft_fs_pu_1v2  "IO8_FT 100MHz fast speed @ 1.2V pullup"
io8_100m_ft_fs_pd_1v2  "IO8_FT 100MHz fast speed @ 1.2V pulldown"
io8_100m_ft_ms_1v2  "IO8_FT 100MHz med speed @ 1.2V"
io8_100m_ft_ms_pu_1v2  "IO8_FT 100MHz med speed @ 1.2V pullup"
io8_100m_ft_ms_pd_1v2  "IO8_FT 100MHz med speed @ 1.2V pulldown"
io8_100m_ft_ls_1v2  "IO8_FT 100MHz low speed @ 1.2V"
io8_100m_ft_ls_pu_1v2  "IO8_FT 100MHz low speed @ 1.2V pullup"
io8_100m_ft_ls_pd_1v2  "IO8_FT 100MHz low speed @ 1.2V pulldown"
io8_100m_ft_hs_1v8  "IO8_FT 100MHz high speed @ 1.8V"
io8_100m_ft_hs_pu_1v8  "IO8_FT 100MHz high speed @ 1.8V pullup"
io8_100m_ft_hs_pd_1v8  "IO8_FT 100MHz high speed @ 1.8V pulldown"
io8_100m_ft_fs_1v8  "IO8_FT 100MHz fast speed @ 1.8V"
io8_100m_ft_fs_pu_1v8  "IO8_FT 100MHz fast speed @ 1.8V pullup"
io8_100m_ft_fs_pd_1v8  "IO8_FT 100MHz fast speed @ 1.8V pulldown"
io8_100m_ft_ms_1v8  "IO8_FT 100MHz med speed @ 1.8V"
io8_100m_ft_ms_pu_1v8  "IO8_FT 100MHz med speed @ 1.8V pullup"
io8_100m_ft_ms_pd_1v8  "IO8_FT 100MHz med speed @ 1.8V pulldown"
io8_100m_ft_ls_1v8  "IO8_FT 100MHz low speed @ 1.8V"
io8_100m_ft_ls_pu_1v8  "IO8_FT 100MHz low speed @ 1.8V pullup"
io8_100m_ft_ls_pd_1v8  "IO8_FT 100MHz low speed @ 1.8V pulldown"
io8_100m_ft_hs_3v3  "IO8_FT 100MHz high speed @ 3.3V"
io8_100m_ft_hs_pu_3v3  "IO8_FT 100MHz high speed @ 3.3V pullup"
io8_100m_ft_hs_pd_3v3  "IO8_FT 100MHz high speed @ 3.3V pulldown"
io8_100m_ft_fs_3v3  "IO8_FT 100MHz fast speed @ 3.3V"
io8_100m_ft_fs_pu_3v3  "IO8_FT 100MHz fast speed @ 3.3V pullup"
io8_100m_ft_fs_pd_3v3  "IO8_FT 100MHz fast speed @ 3.3V pulldown"
io8_100m_ft_ms_3v3  "IO8_FT 100MHz med speed @ 3.3V"
io8_100m_ft_ms_pu_3v3  "IO8_FT 100MHz med speed @ 3.3V pullup"
io8_100m_ft_ms_pd_3v3  "IO8_FT 100MHz med speed @ 3.3V pulldown"
io8_100m_ft_ls_3v3  "IO8_FT 100MHz low speed @ 3.3V"
io8_100m_ft_ls_pu_3v3  "IO8_FT 100MHz low speed @ 3.3V pullup"
io8_100m_ft_ls_pd_3v3  "IO8_FT 100MHz low speed @ 3.3V pulldown"
io8usb_id_nopu  "IOUSB ID @ 3.3V"
io8usb_id_pu  "IOUSB ID @ 3.3V pullup"
[Model Selector] io8_100m_usb_vbus_ft
io8_100m_ft_hs_1v2  "IO8_FT 100MHz high speed @ 1.2V"
io8_100m_ft_hs_pu_1v2  "IO8_FT 100MHz high speed @ 1.2V pullup"
io8_100m_ft_hs_pd_1v2  "IO8_FT 100MHz high speed @ 1.2V pulldown"
io8_100m_ft_fs_1v2  "IO8_FT 100MHz fast speed @ 1.2V"
io8_100m_ft_fs_pu_1v2  "IO8_FT 100MHz fast speed @ 1.2V pullup"
io8_100m_ft_fs_pd_1v2  "IO8_FT 100MHz fast speed @ 1.2V pulldown"
io8_100m_ft_ms_1v2  "IO8_FT 100MHz med speed @ 1.2V"
io8_100m_ft_ms_pu_1v2  "IO8_FT 100MHz med speed @ 1.2V pullup"
io8_100m_ft_ms_pd_1v2  "IO8_FT 100MHz med speed @ 1.2V pulldown"
io8_100m_ft_ls_1v2  "IO8_FT 100MHz low speed @ 1.2V"
io8_100m_ft_ls_pu_1v2  "IO8_FT 100MHz low speed @ 1.2V pullup"
io8_100m_ft_ls_pd_1v2  "IO8_FT 100MHz low speed @ 1.2V pulldown"
io8_100m_ft_hs_1v8  "IO8_FT 100MHz high speed @ 1.8V"
io8_100m_ft_hs_pu_1v8  "IO8_FT 100MHz high speed @ 1.8V pullup"
io8_100m_ft_hs_pd_1v8  "IO8_FT 100MHz high speed @ 1.8V pulldown"
io8_100m_ft_fs_1v8  "IO8_FT 100MHz fast speed @ 1.8V"
io8_100m_ft_fs_pu_1v8  "IO8_FT 100MHz fast speed @ 1.8V pullup"
io8_100m_ft_fs_pd_1v8  "IO8_FT 100MHz fast speed @ 1.8V pulldown"
io8_100m_ft_ms_1v8  "IO8_FT 100MHz med speed @ 1.8V"
io8_100m_ft_ms_pu_1v8  "IO8_FT 100MHz med speed @ 1.8V pullup"
io8_100m_ft_ms_pd_1v8  "IO8_FT 100MHz med speed @ 1.8V pulldown"
io8_100m_ft_ls_1v8  "IO8_FT 100MHz low speed @ 1.8V"
io8_100m_ft_ls_pu_1v8  "IO8_FT 100MHz low speed @ 1.8V pullup"
io8_100m_ft_ls_pd_1v8  "IO8_FT 100MHz low speed @ 1.8V pulldown"
io8_100m_ft_hs_3v3  "IO8_FT 100MHz high speed @ 3.3V"
io8_100m_ft_hs_pu_3v3  "IO8_FT 100MHz high speed @ 3.3V pullup"
io8_100m_ft_hs_pd_3v3  "IO8_FT 100MHz high speed @ 3.3V pulldown"
io8_100m_ft_fs_3v3  "IO8_FT 100MHz fast speed @ 3.3V"
io8_100m_ft_fs_pu_3v3  "IO8_FT 100MHz fast speed @ 3.3V pullup"
io8_100m_ft_fs_pd_3v3  "IO8_FT 100MHz fast speed @ 3.3V pulldown"
io8_100m_ft_ms_3v3  "IO8_FT 100MHz med speed @ 3.3V"
io8_100m_ft_ms_pu_3v3  "IO8_FT 100MHz med speed @ 3.3V pullup"
io8_100m_ft_ms_pd_3v3  "IO8_FT 100MHz med speed @ 3.3V pulldown"
io8_100m_ft_ls_3v3  "IO8_FT 100MHz low speed @ 3.3V"
io8_100m_ft_ls_pu_3v3  "IO8_FT 100MHz low speed @ 3.3V pullup"
io8_100m_ft_ls_pd_3v3  "IO8_FT 100MHz low speed @ 3.3V pulldown"
io8usb_adp "IOUSB ADP @ 3.3V"
io8usb_vbus "IOUSB VBUS @ 3.3V"
[Model Selector] io8_166m_hslv_ft
io8_166m_ft_hs_1v2  "IO8_FT 166MHz high speed @ 1.2V"
io8_166m_ft_hs_pu_1v2  "IO8_FT 166MHz high speed @ 1.2V pullup"
io8_166m_ft_hs_pd_1v2  "IO8_FT 166MHz high speed @ 1.2V pulldown"
io8_166m_ft_fs_1v2  "IO8_FT 166MHz fast speed @ 1.2V"
io8_166m_ft_fs_pu_1v2  "IO8_FT 166MHz fast speed @ 1.2V pullup"
io8_166m_ft_fs_pd_1v2  "IO8_FT 166MHz fast speed @ 1.2V pulldown"
io8_166m_ft_ms_1v2  "IO8_FT 166MHz med speed @ 1.2V"
io8_166m_ft_ms_pu_1v2  "IO8_FT 166MHz med speed @ 1.2V pullup"
io8_166m_ft_ms_pd_1v2  "IO8_FT 166MHz med speed @ 1.2V pulldown"
io8_166m_ft_ls_1v2  "IO8_FT 166MHz low speed @ 1.2V"
io8_166m_ft_ls_pu_1v2  "IO8_FT 166MHz low speed @ 1.2V pullup"
io8_166m_ft_ls_pd_1v2  "IO8_FT 166MHz low speed @ 1.2V pulldown"
io8_166m_ft_hs_1v8  "IO8_FT 166MHz high speed @ 1.8V"
io8_166m_ft_hs_pu_1v8  "IO8_FT 166MHz high speed @ 1.8V pullup"
io8_166m_ft_hs_pd_1v8  "IO8_FT 166MHz high speed @ 1.8V pulldown"
io8_166m_ft_fs_1v8  "IO8_FT 166MHz fast speed @ 1.8V"
io8_166m_ft_fs_pu_1v8  "IO8_FT 166MHz fast speed @ 1.8V pullup"
io8_166m_ft_fs_pd_1v8  "IO8_FT 166MHz fast speed @ 1.8V pulldown"
io8_166m_ft_ms_1v8  "IO8_FT 166MHz med speed @ 1.8V"
io8_166m_ft_ms_pu_1v8  "IO8_FT 166MHz med speed @ 1.8V pullup"
io8_166m_ft_ms_pd_1v8  "IO8_FT 166MHz med speed @ 1.8V pulldown"
io8_166m_ft_ls_1v8  "IO8_FT 166MHz low speed @ 1.8V"
io8_166m_ft_ls_pu_1v8  "IO8_FT 166MHz low speed @ 1.8V pullup"
io8_166m_ft_ls_pd_1v8  "IO8_FT 166MHz low speed @ 1.8V pulldown"
io8_166m_ft_hs_3v3  "IO8_FT 166MHz high speed @ 3.3V"
io8_166m_ft_hs_pu_3v3  "IO8_FT 166MHz high speed @ 3.3V pullup"
io8_166m_ft_hs_pd_3v3  "IO8_FT 166MHz high speed @ 3.3V pulldown"
io8_166m_ft_fs_3v3  "IO8_FT 166MHz fast speed @ 3.3V"
io8_166m_ft_fs_pu_3v3  "IO8_FT 166MHz fast speed @ 3.3V pullup"
io8_166m_ft_fs_pd_3v3  "IO8_FT 166MHz fast speed @ 3.3V pulldown"
io8_166m_ft_ms_3v3  "IO8_FT 166MHz med speed @ 3.3V"
io8_166m_ft_ms_pu_3v3  "IO8_FT 166MHz med speed @ 3.3V pullup"
io8_166m_ft_ms_pd_3v3  "IO8_FT 166MHz med speed @ 3.3V pulldown"
io8_166m_ft_ls_3v3  "IO8_FT 166MHz low speed @ 3.3V"
io8_166m_ft_ls_pu_3v3  "IO8_FT 166MHz low speed @ 3.3V pullup"
io8_166m_ft_ls_pd_3v3  "IO8_FT 166MHz low speed @ 3.3V pulldown"
io8_166m_hslv_ft_hs_1v2  "IO8_FT 166MHz HSLV high speed @ 1.2V"
io8_166m_hslv_ft_hs_pu_1v2  "IO8_FT 166MHz HSLV high speed @ 1.2V pullup"
io8_166m_hslv_ft_hs_pd_1v2  "IO8_FT 166MHz HSLV high speed @ 1.2V pulldown"
io8_166m_hslv_ft_fs_1v2  "IO8_FT 166MHz HSLV fast speed @ 1.2V"
io8_166m_hslv_ft_fs_pu_1v2  "IO8_FT 166MHz HSLV fast speed @ 1.2V pullup"
io8_166m_hslv_ft_fs_pd_1v2  "IO8_FT 166MHz HSLV fast speed @ 1.2V pulldown"
io8_166m_hslv_ft_ms_1v2  "IO8_FT 166MHz HSLV med speed @ 1.2V"
io8_166m_hslv_ft_ms_pu_1v2  "IO8_FT 166MHz HSLV med speed @ 1.2V pullup"
io8_166m_hslv_ft_ms_pd_1v2  "IO8_FT 166MHz HSLV med speed @ 1.2V pulldown"
io8_166m_hslv_ft_ls_1v2  "IO8_FT 166MHz HSLV low speed @ 1.2V"
io8_166m_hslv_ft_ls_pu_1v2  "IO8_FT 166MHz HSLV low speed @ 1.2V pullup"
io8_166m_hslv_ft_ls_pd_1v2  "IO8_FT 166MHz HSLV low speed @ 1.2V pulldown"
io8_166m_hslv_ft_hs_1v8  "IO8_FT 166MHz HSLV high speed @ 1.8V"
io8_166m_hslv_ft_hs_pu_1v8  "IO8_FT 166MHz HSLV high speed @ 1.8V pullup"
io8_166m_hslv_ft_hs_pd_1v8  "IO8_FT 166MHz HSLV high speed @ 1.8V pulldown"
io8_166m_hslv_ft_fs_1v8  "IO8_FT 166MHz HSLV fast speed @ 1.8V"
io8_166m_hslv_ft_fs_pu_1v8  "IO8_FT 166MHz HSLV fast speed @ 1.8V pullup"
io8_166m_hslv_ft_fs_pd_1v8  "IO8_FT 166MHz HSLV fast speed @ 1.8V pulldown"
io8_166m_hslv_ft_ms_1v8  "IO8_FT 166MHz HSLV med speed @ 1.8V"
io8_166m_hslv_ft_ms_pu_1v8  "IO8_FT 166MHz HSLV med speed @ 1.8V pullup"
io8_166m_hslv_ft_ms_pd_1v8  "IO8_FT 166MHz HSLV med speed @ 1.8V pulldown"
io8_166m_hslv_ft_ls_1v8  "IO8_FT 166MHz HSLV low speed @ 1.8V"
io8_166m_hslv_ft_ls_pu_1v8  "IO8_FT 166MHz HSLV low speed @ 1.8V pullup"
io8_166m_hslv_ft_ls_pd_1v8  "IO8_FT 166MHz HSLV low speed @ 1.8V pulldown"
io8_166m_hslv_ft_hs_2v5  "IO8_FT 166MHz HSLV high speed @ 2.5V"
io8_166m_hslv_ft_hs_pu_2v5  "IO8_FT 166MHz HSLV high speed @ 2.5V pullup"
io8_166m_hslv_ft_hs_pd_2v5  "IO8_FT 166MHz HSLV high speed @ 2.5V pulldown"
io8_166m_hslv_ft_fs_2v5  "IO8_FT 166MHz HSLV fast speed @ 2.5V"
io8_166m_hslv_ft_fs_pu_2v5  "IO8_FT 166MHz HSLV fast speed @ 2.5V pullup"
io8_166m_hslv_ft_fs_pd_2v5  "IO8_FT 166MHz HSLV fast speed @ 2.5V pulldown"
io8_166m_hslv_ft_ms_2v5  "IO8_FT 166MHz HSLV med speed @ 2.5V"
io8_166m_hslv_ft_ms_pu_2v5  "IO8_FT 166MHz HSLV med speed @ 2.5V pullup"
io8_166m_hslv_ft_ms_pd_2v5  "IO8_FT 166MHz HSLV med speed @ 2.5V pulldown"
io8_166m_hslv_ft_ls_2v5  "IO8_FT 166MHz HSLV low speed @ 2.5V"
io8_166m_hslv_ft_ls_pu_2v5  "IO8_FT 166MHz HSLV low speed @ 2.5V pullup"
io8_166m_hslv_ft_ls_pd_2v5  "IO8_FT 166MHz HSLV low speed @ 2.5V pulldown"
[Model Selector] io8_spi_hslv_ft
io8_spi_ft_hs_1v2  "IO8_FT SPI high speed @ 1.2V"
io8_spi_ft_hs_pu_1v2  "IO8_FT SPI high speed @ 1.2V pullup"
io8_spi_ft_hs_pd_1v2  "IO8_FT SPI high speed @ 1.2V pulldown"
io8_spi_ft_fs_1v2  "IO8_FT SPI fast speed @ 1.2V"
io8_spi_ft_fs_pu_1v2  "IO8_FT SPI fast speed @ 1.2V pullup"
io8_spi_ft_fs_pd_1v2  "IO8_FT SPI fast speed @ 1.2V pulldown"
io8_spi_ft_ms_1v2  "IO8_FT SPI med speed @ 1.2V"
io8_spi_ft_ms_pu_1v2  "IO8_FT SPI med speed @ 1.2V pullup"
io8_spi_ft_ms_pd_1v2  "IO8_FT SPI med speed @ 1.2V pulldown"
io8_spi_ft_ls_1v2  "IO8_FT SPI low speed @ 1.2V"
io8_spi_ft_ls_pu_1v2  "IO8_FT SPI low speed @ 1.2V pullup"
io8_spi_ft_ls_pd_1v2  "IO8_FT SPI low speed @ 1.2V pulldown"
io8_spi_ft_hs_1v8  "IO8_FT SPI high speed @ 1.8V"
io8_spi_ft_hs_pu_1v8  "IO8_FT SPI high speed @ 1.8V pullup"
io8_spi_ft_hs_pd_1v8  "IO8_FT SPI high speed @ 1.8V pulldown"
io8_spi_ft_fs_1v8  "IO8_FT SPI fast speed @ 1.8V"
io8_spi_ft_fs_pu_1v8  "IO8_FT SPI fast speed @ 1.8V pullup"
io8_spi_ft_fs_pd_1v8  "IO8_FT SPI fast speed @ 1.8V pulldown"
io8_spi_ft_ms_1v8  "IO8_FT SPI med speed @ 1.8V"
io8_spi_ft_ms_pu_1v8  "IO8_FT SPI med speed @ 1.8V pullup"
io8_spi_ft_ms_pd_1v8  "IO8_FT SPI med speed @ 1.8V pulldown"
io8_spi_ft_ls_1v8  "IO8_FT SPI low speed @ 1.8V"
io8_spi_ft_ls_pu_1v8  "IO8_FT SPI low speed @ 1.8V pullup"
io8_spi_ft_ls_pd_1v8  "IO8_FT SPI low speed @ 1.8V pulldown"
io8_spi_ft_hs_3v3  "IO8_FT SPI high speed @ 3.3V"
io8_spi_ft_hs_pu_3v3  "IO8_FT SPI high speed @ 3.3V pullup"
io8_spi_ft_hs_pd_3v3  "IO8_FT SPI high speed @ 3.3V pulldown"
io8_spi_ft_fs_3v3  "IO8_FT SPI fast speed @ 3.3V"
io8_spi_ft_fs_pu_3v3  "IO8_FT SPI fast speed @ 3.3V pullup"
io8_spi_ft_fs_pd_3v3  "IO8_FT SPI fast speed @ 3.3V pulldown"
io8_spi_ft_ms_3v3  "IO8_FT SPI med speed @ 3.3V"
io8_spi_ft_ms_pu_3v3  "IO8_FT SPI med speed @ 1.8V pullup"
io8_spi_ft_ms_pd_3v3  "IO8_FT SPI med speed @ 3.3V pulldown"
io8_spi_ft_ls_3v3  "IO8_FT SPI low speed @ 3.3V"
io8_spi_ft_ls_pu_3v3  "IO8_FT SPI low speed @ 3.3V pullup"
io8_spi_ft_ls_pd_3v3  "IO8_FT SPI low speed @ 3.3V pulldown"
io8_spi_hslv_ft_hs_1v2  "IO8_FT SPI HSLV high speed @ 1.2V"
io8_spi_hslv_ft_hs_pu_1v2  "IO8_FT SPI HSLV high speed @ 1.2V pullup"
io8_spi_hslv_ft_hs_pd_1v2  "IO8_FT SPI HSLV high speed @ 1.2V pulldown"
io8_spi_hslv_ft_fs_1v2  "IO8_FT SPI HSLV fast speed @ 1.2V"
io8_spi_hslv_ft_fs_pu_1v2  "IO8_FT SPI HSLV fast speed @ 1.2V pullup"
io8_spi_hslv_ft_fs_pd_1v2  "IO8_FT SPI HSLV fast speed @ 1.2V pulldown"
io8_spi_hslv_ft_ms_1v2  "IO8_FT SPI HSLV med speed @ 1.2V"
io8_spi_hslv_ft_ms_pu_1v2  "IO8_FT SPI HSLV med speed @ 1.2V pullup"
io8_spi_hslv_ft_ms_pd_1v2  "IO8_FT SPI HSLV med speed @ 1.2V pulldown"
io8_spi_hslv_ft_ls_1v2  "IO8_FT SPI HSLV low speed @ 1.2V"
io8_spi_hslv_ft_ls_pu_1v2  "IO8_FT SPI HSLV low speed @ 1.2V pullup"
io8_spi_hslv_ft_ls_pd_1v2  "IO8_FT SPI HSLV low speed @ 1.2V pulldown"
io8_spi_hslv_ft_hs_1v8  "IO8_FT SPI HSLV high speed @ 1.8V"
io8_spi_hslv_ft_hs_pu_1v8  "IO8_FT SPI HSLV high speed @ 1.8V pullup"
io8_spi_hslv_ft_hs_pd_1v8  "IO8_FT SPI HSLV high speed @ 1.8V pulldown"
io8_spi_hslv_ft_fs_1v8  "IO8_FT SPI HSLV fast speed @ 1.8V"
io8_spi_hslv_ft_fs_pu_1v8  "IO8_FT SPI HSLV fast speed @ 1.8V pullup"
io8_spi_hslv_ft_fs_pd_1v8  "IO8_FT SPI HSLV fast speed @ 1.8V pulldown"
io8_spi_hslv_ft_ms_1v8  "IO8_FT SPI HSLV med speed @ 1.8V"
io8_spi_hslv_ft_ms_pu_1v8  "IO8_FT SPI HSLV med speed @ 1.8V pullup"
io8_spi_hslv_ft_ms_pd_1v8  "IO8_FT SPI HSLV med speed @ 1.8V pulldown"
io8_spi_hslv_ft_ls_1v8  "IO8_FT SPI HSLV low speed @ 1.8V"
io8_spi_hslv_ft_ls_pu_1v8  "IO8_FT SPI HSLV low speed @ 1.8V pullup"
io8_spi_hslv_ft_ls_pd_1v8  "IO8_FT SPI HSLV low speed @ 1.8V pulldown"
io8_spi_hslv_ft_hs_2v5  "IO8_FT SPI HSLV high speed @ 2.5V"
io8_spi_hslv_ft_hs_pu_2v5  "IO8_FT SPI HSLV high speed @ 2.5V pullup"
io8_spi_hslv_ft_hs_pd_2v5  "IO8_FT SPI HSLV high speed @ 2.5V pulldown"
io8_spi_hslv_ft_fs_2v5  "IO8_FT SPI HSLV fast speed @ 2.5V"
io8_spi_hslv_ft_fs_pu_2v5  "IO8_FT SPI HSLV fast speed @ 2.5V pullup"
io8_spi_hslv_ft_fs_pd_2v5  "IO8_FT SPI HSLV fast speed @ 2.5V pulldown"
io8_spi_hslv_ft_ms_2v5  "IO8_FT SPI HSLV med speed @ 2.5V"
io8_spi_hslv_ft_ms_pu_2v5  "IO8_FT SPI HSLV med speed @ 2.5V pullup"
io8_spi_hslv_ft_ms_pd_2v5  "IO8_FT SPI HSLV med speed @ 2.5V pulldown"
io8_spi_hslv_ft_ls_2v5  "IO8_FT SPI HSLV low speed @ 2.5V"
io8_spi_hslv_ft_ls_pu_2v5  "IO8_FT SPI HSLV low speed @ 2.5V pullup"
io8_spi_hslv_ft_ls_pd_2v5  "IO8_FT SPI HSLV low speed @ 2.5V pulldown"
[Model Selector] io8_spi_ft
io8_spi_ft_hs_1v2  "IO8_FT SPI high speed @ 1.2V"
io8_spi_ft_hs_pu_1v2  "IO8_FT SPI high speed @ 1.2V pullup"
io8_spi_ft_hs_pd_1v2  "IO8_FT SPI high speed @ 1.2V pulldown"
io8_spi_ft_fs_1v2  "IO8_FT SPI fast speed @ 1.2V"
io8_spi_ft_fs_pu_1v2  "IO8_FT SPI fast speed @ 1.2V pullup"
io8_spi_ft_fs_pd_1v2  "IO8_FT SPI fast speed @ 1.2V pulldown"
io8_spi_ft_ms_1v2  "IO8_FT SPI med speed @ 1.2V"
io8_spi_ft_ms_pu_1v2  "IO8_FT SPI med speed @ 1.2V pullup"
io8_spi_ft_ms_pd_1v2  "IO8_FT SPI med speed @ 1.2V pulldown"
io8_spi_ft_ls_1v2  "IO8_FT SPI low speed @ 1.2V"
io8_spi_ft_ls_pu_1v2  "IO8_FT SPI low speed @ 1.2V pullup"
io8_spi_ft_ls_pd_1v2  "IO8_FT SPI low speed @ 1.2V pulldown"
io8_spi_ft_hs_1v8  "IO8_FT SPI high speed @ 1.8V"
io8_spi_ft_hs_pu_1v8  "IO8_FT SPI high speed @ 1.8V pullup"
io8_spi_ft_hs_pd_1v8  "IO8_FT SPI high speed @ 1.8V pulldown"
io8_spi_ft_fs_1v8  "IO8_FT SPI fast speed @ 1.8V"
io8_spi_ft_fs_pu_1v8  "IO8_FT SPI fast speed @ 1.8V pullup"
io8_spi_ft_fs_pd_1v8  "IO8_FT SPI fast speed @ 1.8V pulldown"
io8_spi_ft_ms_1v8  "IO8_FT SPI med speed @ 1.8V"
io8_spi_ft_ms_pu_1v8  "IO8_FT SPI med speed @ 1.8V pullup"
io8_spi_ft_ms_pd_1v8  "IO8_FT SPI med speed @ 1.8V pulldown"
io8_spi_ft_ls_1v8  "IO8_FT SPI low speed @ 1.8V"
io8_spi_ft_ls_pu_1v8  "IO8_FT SPI low speed @ 1.8V pullup"
io8_spi_ft_ls_pd_1v8  "IO8_FT SPI low speed @ 1.8V pulldown"
io8_spi_ft_hs_3v3  "IO8_FT SPI high speed @ 3.3V"
io8_spi_ft_hs_pu_3v3  "IO8_FT SPI high speed @ 3.3V pullup"
io8_spi_ft_hs_pd_3v3  "IO8_FT SPI high speed @ 3.3V pulldown"
io8_spi_ft_fs_3v3  "IO8_FT SPI fast speed @ 3.3V"
io8_spi_ft_fs_pu_3v3  "IO8_FT SPI fast speed @ 3.3V pullup"
io8_spi_ft_fs_pd_3v3  "IO8_FT SPI fast speed @ 3.3V pulldown"
io8_spi_ft_ms_3v3  "IO8_FT SPI med speed @ 3.3V"
io8_spi_ft_ms_pu_3v3  "IO8_FT SPI med speed @ 1.8V pullup"
io8_spi_ft_ms_pd_3v3  "IO8_FT SPI med speed @ 3.3V pulldown"
io8_spi_ft_ls_3v3  "IO8_FT SPI low speed @ 3.3V"
io8_spi_ft_ls_pu_3v3  "IO8_FT SPI low speed @ 3.3V pullup"
io8_spi_ft_ls_pd_3v3  "IO8_FT SPI low speed @ 3.3V pulldown"
io8_spi_hslv_ft_hs_1v2  "IO8_FT SPI HSLV high speed @ 1.2V"
io8_spi_hslv_ft_hs_pu_1v2  "IO8_FT SPI HSLV high speed @ 1.2V pullup"
io8_spi_hslv_ft_hs_pd_1v2  "IO8_FT SPI HSLV high speed @ 1.2V pulldown"
io8_spi_hslv_ft_fs_1v2  "IO8_FT SPI HSLV fast speed @ 1.2V"
io8_spi_hslv_ft_fs_pu_1v2  "IO8_FT SPI HSLV fast speed @ 1.2V pullup"
io8_spi_hslv_ft_fs_pd_1v2  "IO8_FT SPI HSLV fast speed @ 1.2V pulldown"
io8_spi_hslv_ft_ms_1v2  "IO8_FT SPI HSLV med speed @ 1.2V"
io8_spi_hslv_ft_ms_pu_1v2  "IO8_FT SPI HSLV med speed @ 1.2V pullup"
io8_spi_hslv_ft_ms_pd_1v2  "IO8_FT SPI HSLV med speed @ 1.2V pulldown"
io8_spi_hslv_ft_ls_1v2  "IO8_FT SPI HSLV low speed @ 1.2V"
io8_spi_hslv_ft_ls_pu_1v2  "IO8_FT SPI HSLV low speed @ 1.2V pullup"
io8_spi_hslv_ft_ls_pd_1v2  "IO8_FT SPI HSLV low speed @ 1.2V pulldown"
io8_spi_hslv_ft_hs_1v8  "IO8_FT SPI HSLV high speed @ 1.8V"
io8_spi_hslv_ft_hs_pu_1v8  "IO8_FT SPI HSLV high speed @ 1.8V pullup"
io8_spi_hslv_ft_hs_pd_1v8  "IO8_FT SPI HSLV high speed @ 1.8V pulldown"
io8_spi_hslv_ft_fs_1v8  "IO8_FT SPI HSLV fast speed @ 1.8V"
io8_spi_hslv_ft_fs_pu_1v8  "IO8_FT SPI HSLV fast speed @ 1.8V pullup"
io8_spi_hslv_ft_fs_pd_1v8  "IO8_FT SPI HSLV fast speed @ 1.8V pulldown"
io8_spi_hslv_ft_ms_1v8  "IO8_FT SPI HSLV med speed @ 1.8V"
io8_spi_hslv_ft_ms_pu_1v8  "IO8_FT SPI HSLV med speed @ 1.8V pullup"
io8_spi_hslv_ft_ms_pd_1v8  "IO8_FT SPI HSLV med speed @ 1.8V pulldown"
io8_spi_hslv_ft_ls_1v8  "IO8_FT SPI HSLV low speed @ 1.8V"
io8_spi_hslv_ft_ls_pu_1v8  "IO8_FT SPI HSLV low speed @ 1.8V pullup"
io8_spi_hslv_ft_ls_pd_1v8  "IO8_FT SPI HSLV low speed @ 1.8V pulldown"
io8_spi_hslv_ft_hs_2v5  "IO8_FT SPI HSLV high speed @ 2.5V"
io8_spi_hslv_ft_hs_pu_2v5  "IO8_FT SPI HSLV high speed @ 2.5V pullup"
io8_spi_hslv_ft_hs_pd_2v5  "IO8_FT SPI HSLV high speed @ 2.5V pulldown"
io8_spi_hslv_ft_fs_2v5  "IO8_FT SPI HSLV fast speed @ 2.5V"
io8_spi_hslv_ft_fs_pu_2v5  "IO8_FT SPI HSLV fast speed @ 2.5V pullup"
io8_spi_hslv_ft_fs_pd_2v5  "IO8_FT SPI HSLV fast speed @ 2.5V pulldown"
io8_spi_hslv_ft_ms_2v5  "IO8_FT SPI HSLV med speed @ 2.5V"
io8_spi_hslv_ft_ms_pu_2v5  "IO8_FT SPI HSLV med speed @ 2.5V pullup"
io8_spi_hslv_ft_ms_pd_2v5  "IO8_FT SPI HSLV med speed @ 2.5V pulldown"
io8_spi_hslv_ft_ls_2v5  "IO8_FT SPI HSLV low speed @ 2.5V"
io8_spi_hslv_ft_ls_pu_2v5  "IO8_FT SPI HSLV low speed @ 2.5V pullup"
io8_spi_hslv_ft_ls_pd_2v5  "IO8_FT SPI HSLV low speed @ 2.5V pulldown"
[Define Package Model]  481-wlcsp-208-221128
[Manufacturer]  Unknown
[OEM]  Unknown
[Description]  None
[Number Of Pins]  180
[Pin Numbers]
| Pin Num   Terminal Name
H25 | DSI_CKN
G26 | DSI_CKP
F25 | DSI_D0N
E26 | DSI_D0P
K25 | DSI_D1N
J26 | DSI_D1P
M21 | NRST
N22 | PA0
L16 | PA1
M17 | PA2
P23 | PA3
N20 | PA4
P21 | PA5
N18 | PA6
R22 | PA7
C8 | PA8
C6 | PA9
C4 | PA10
C2 | PA11
B1 | PA12
B3 | PA13
D11 | PA14
A8 | PA15
H13 | PB0
L14 | PB1
M15 | PB2
B17 | PB3
G18 | PB4
C18 | PB5
A18 | PB6
D19 | PB7
B19 | PB8
C20 | PB9
T13 | PB10
R10 | PB11
T5 | PB12
T7 | PB13
R6 | PB14
P11 | PB15
K17 | PC0
K15 | PC1
L18 | PC2
M19 | PC3
T23 | PC4
P19 | PC5
D5 | PC6
D3 | PC7
D7 | PC8
D9 | PC9
B9 | PC10
C10 | PC11
E14 | PC12
D23 | PC13
C26 | PC14-OSC32_IN
D25 | PC15-OSC32_OUT
F15 | PD0
A10 | PD1
D13 | PD2
C12 | PD3
D15 | PD4
E16 | PD5
F17 | PD6
C14 | PD7
P9 | PD8
P7 | PD9
P5 | PD10
M11 | PD11
L10 | PD12
K11 | PD13
N10 | PD14
K9 | PD15
A20 | PE0
B21 | PE1
G20 | PE2
E22 | PE3
F21 | PE4
G22 | PE5
C24 | PE6
L12 | PE7
N14 | PE8
T17 | PE9
M13 | PE10
P15 | PE11
R14 | PE12
N12 | PE13
P13 | PE14
R12 | PE15
H19 | PF0
H21 | PF1
J20 | PF2
K23 | PF3
J22 | PF4
K21 | PF5
J16 | PF6
J14 | PF7
K19 | PF8
L20 | PF9
L22 | PF10
N16 | PF11
T21 | PF12
P17 | PF13
K13 | PF14
R18 | PF15
H11 | PG0
J12 | PG1
F9 | PG2
H9 | PG3
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| Models and submodels in the file (265): io8_100m_ft_hs_1v2 (I/O), io8_100m_ft_hs_pu_1v2 (I/O), io8_100m_ft_hs_pd_1v2 (I/O), io8_100m_ft_fs_1v2 (I/O), io8_100m_ft_fs_pu_1v2 (I/O), io8_100m_ft_fs_pd_1v2 (I/O), io8_100m_ft_ms_1v2 (I/O), io8_100m_ft_ms_pu_1v2 (I/O), io8_100m_ft_ms_pd_1v2 (I/O), io8_100m_ft_ls_1v2 (I/O), io8_100m_ft_ls_pu_1v2 (I/O), io8_100m_ft_ls_pd_1v2 (I/O), io8_100m_ft_hs_1v8 (I/O), io8_100m_ft_hs_pu_1v8 (I/O), io8_100m_ft_hs_pd_1v8 (I/O), io8_100m_ft_fs_1v8 (I/O), io8_100m_ft_fs_pu_1v8 (I/O), io8_100m_ft_fs_pd_1v8 (I/O), io8_100m_ft_ms_1v8 (I/O), io8_100m_ft_ms_pu_1v8 (I/O), io8_100m_ft_ms_pd_1v8 (I/O), io8_100m_ft_ls_1v8 (I/O), io8_100m_ft_ls_pu_1v8 (I/O), io8_100m_ft_ls_pd_1v8 (I/O), io8_100m_ft_hs_3v3 (I/O), io8_100m_ft_hs_pu_3v3 (I/O), io8_100m_ft_hs_pd_3v3 (I/O), io8_100m_ft_fs_3v3 (I/O), io8_100m_ft_fs_pu_3v3 (I/O), io8_100m_ft_fs_pd_3v3 (I/O), io8_100m_ft_ms_3v3 (I/O), io8_100m_ft_ms_pu_3v3 (I/O), io8_100m_ft_ms_pd_3v3 (I/O), io8_100m_ft_ls_3v3 (I/O), io8_100m_ft_ls_pu_3v3 (I/O), io8_100m_ft_ls_pd_3v3 (I/O), io8_100m_hslv_ft_hs_1v2 (I/O), io8_100m_hslv_ft_hs_pu_1v2 (I/O), io8_100m_hslv_ft_hs_pd_1v2 (I/O), io8_100m_hslv_ft_fs_1v2 (I/O), io8_100m_hslv_ft_fs_pu_1v2 (I/O), io8_100m_hslv_ft_fs_pd_1v2 (I/O), io8_100m_hslv_ft_ms_1v2 (I/O), io8_100m_hslv_ft_ms_pu_1v2 (I/O), io8_100m_hslv_ft_ms_pd_1v2 (I/O), io8_100m_hslv_ft_ls_1v2 (I/O), io8_100m_hslv_ft_ls_pu_1v2 (I/O), io8_100m_hslv_ft_ls_pd_1v2 (I/O), io8_100m_hslv_ft_hs_1v8 (I/O), io8_100m_hslv_ft_hs_pu_1v8 (I/O), io8_100m_hslv_ft_hs_pd_1v8 (I/O), io8_100m_hslv_ft_fs_1v8 (I/O), io8_100m_hslv_ft_fs_pu_1v8 (I/O), io8_100m_hslv_ft_fs_pd_1v8 (I/O), io8_100m_hslv_ft_ms_1v8 (I/O), io8_100m_hslv_ft_ms_pu_1v8 (I/O), io8_100m_hslv_ft_ms_pd_1v8 (I/O), io8_100m_hslv_ft_ls_1v8 (I/O), io8_100m_hslv_ft_ls_pu_1v8 (I/O), io8_100m_hslv_ft_ls_pd_1v8 (I/O), io8_100m_hslv_ft_hs_2v5 (I/O), io8_100m_hslv_ft_hs_pu_2v5 (I/O), io8_100m_hslv_ft_hs_pd_2v5 (I/O), io8_100m_hslv_ft_fs_2v5 (I/O), io8_100m_hslv_ft_fs_pu_2v5 (I/O), io8_100m_hslv_ft_fs_pd_2v5 (I/O), io8_100m_hslv_ft_ms_2v5 (I/O), io8_100m_hslv_ft_ms_pu_2v5 (I/O), io8_100m_hslv_ft_ms_pd_2v5 (I/O), io8_100m_hslv_ft_ls_2v5 (I/O), io8_100m_hslv_ft_ls_pu_2v5 (I/O), io8_100m_hslv_ft_ls_pd_2v5 (I/O), io8_100m_i2c_ft_1v2 (I/O_open_drain), io8_100m_i2c_ft_pu_1v2 (I/O_open_drain), io8_100m_i2c_ft_pd_1v2 (I/O_open_drain), io8_100m_i2c_ft_1v8 (I/O_open_drain), io8_100m_i2c_ft_pu_1v8 (I/O_open_drain), io8_100m_i2c_ft_pd_1v8 (I/O_open_drain), io8_100m_i2c_ft_3v3 (I/O_open_drain), io8_100m_i2c_ft_pu_3v3 (I/O_open_drain)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
